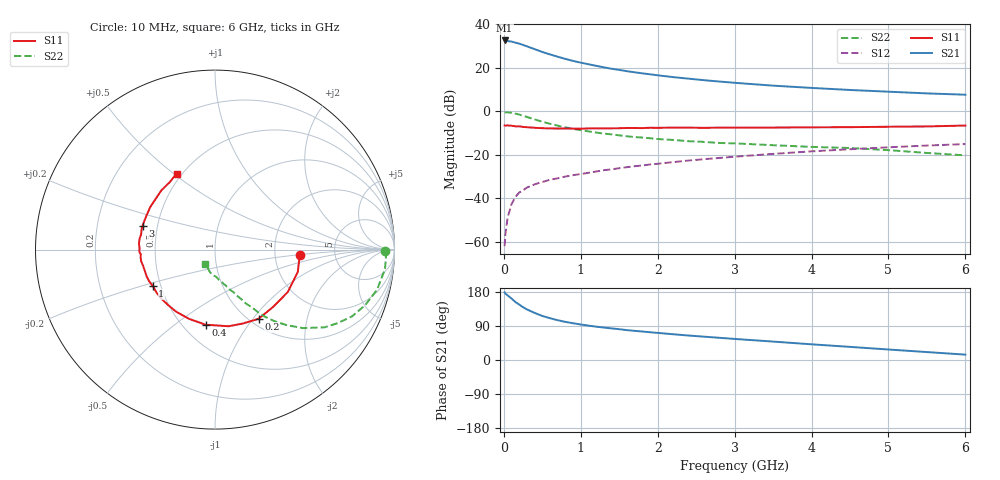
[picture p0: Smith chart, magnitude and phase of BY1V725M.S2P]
! SIEMENS Small Signal Semiconductors
! BFY420
! Si NPN RF SIEGET Grounded Emitter Transistor in MICRO-X
! VCE = 1.75 V  IC = 25 mA
! Common Emitter S-Parameters:  October  1996
# GHz  S  MA  R  50
!  f  S11  S21  S12  S22
! GHz  MAG  ANG  MAG  ANG  MAG  ANG  MAG  ANG
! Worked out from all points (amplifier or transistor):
!   36 points, 10 MHz to 6 GHz, reference 50 ohm
!   highest |S21| = 32.6 dB at 10 MHz (marker M1)
!   |S21| within 3 dB of that: start of sweep to 323.2 MHz
!   unconditionally stable (mu >= 1): 1.717 GHz to end of sweep
!   at 250 MHz: K = 0.34, MSG = 33.4 dB, |S12| = -36.2 dB
!   at 1.4 GHz: K = 0.95, MSG = 23.1 dB, |S12| = -26.6 dB
!   at 6 GHz: K = 1.07, MAG = 9.7 dB, |S12| = -15.0 dB
!   S11 on the Smith chart (normalised r, x): 10 MHz: 2.80, -0.22; 200 MHz: 1.10, -1.07; 400 MHz: 0.64, -0.65; 1 GHz: 0.45, -0.22; 3 GHz: 0.41, +0.13; 6 GHz: 0.47, +0.51
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0.01  0.4763 -3.7  42.86 178.5  0.0008 109.0  0.9478 -0.6
0.02  0.4726 -6.7  42.74 175.4  0.0015 86.0  0.9536 -2.1
0.1  0.4696 -30.2  40.36 162.2  0.0074 80.1  0.9302 -13.9
0.15  0.4548 -44.3  38.24 153.1  0.0108 73.3  0.8916 -20.4
0.2  0.4559 -57.7  36.21 146.3  0.0137 70.7  0.8491 -26.0
0.25  0.4401 -69.3  33.79 139.2  0.0154 67.1  0.7951 -31.1
0.3  0.4339 -79.9  31.4 133.5  0.0178 65.1  0.7479 -35.4
0.4  0.4217 -97.2  27.09 124.3  0.0211 61.5  0.656 -41.8
0.5  0.412 -110.9  23.29 116.3  0.0239 59.6  0.5803 -46.5
0.6  0.408 -122.3  20.48 110.3  0.0269 58.3  0.5198 -50.2
0.7  0.4046 -130.7  18.14 105.0  0.029 58.5  0.4716 -53.0
0.8  0.4052 -137.9  16.13 100.6  0.0319 57.7  0.4307 -55.2
1  0.4019 -149.7  13.23 93.7  0.0364 58.1  0.3716 -58.2
1.1  0.4071 -154.5  12.17 90.7  0.0389 58.9  0.3483 -60.0
1.4  0.4098 -165.8  9.585 83.4  0.0466 58.8  0.2969 -63.4
1.6  0.4169 -171.1  8.429 78.8  0.0524 58.8  0.2689 -65.8
2.2  0.4252 175.4  6.158 68.0  0.0684 56.6  0.2212 -71.8
3  0.4252 161.8  4.558 55.6  0.0912 52.1  0.1847 -78.7
3.5  0.4262 153.8  3.921 48.6  0.1059 48.5  0.1675 -83.3
4.5  0.4352 139.2  3.117 34.6  0.1352 40.2  0.1444 -92.6
5.5  0.4525 123.8  2.601 20.9  0.1645 30.5  0.1111 -111.0
6  0.4741 116.9  2.427 14.2  0.1779 25.5  0.0978 -125.5
